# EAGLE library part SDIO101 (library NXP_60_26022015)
SD/SDIO/MMC/CE-ATA host controller The SDIO101 is a SD/SDIO/MMC/CE-ATA host controller with a standard 16-bit asynchronous memory interface. The device conforms to the SD Host Standard Specification Version 2.0. The SDIO101 manages the physical layer of SD, SDIO, MMC and CE-ATA protocols and can be used together with SD Host Standard compatible driver software to add SD/SDIO/MMC/CE-ATA host functionality to a variety of microprocessor systems. The SDIO101 supports both full-speed (lower than 25 MHz) and high-speed (lower than 52 MHz) data transmissions on the SD/SDIO/MMC/CE-ATA port. The SDIO101 offers separate pins for SD/SDIO/MMC/CE-ATA port supply voltage, host interface supply voltage and core supply voltage. The SD/SDIO/MMC/CE-ATA port can operate at a wide voltage range (1.8 V to 3.6 V) which allows the device to interface to a large variety of SD, SDIO, MMC or CE-ATA devices. The SDIO101 allows 1-bit and 4-bit SD transactions and 8-bit MMC/CE-ATA transactions. The 16-bit asynchronous memory interface can operate at a 2.5 V to 3.6 V voltage range. A built-in, 2 kB data buffer allows for a low interrupt latency time and efficient communication with the host processor at high data rates. The SDIO101 provides a DMA request line that can be connected to an external DMA controller to off-load the host processor and increase overall system performance. An on-board PLL allows a large range of SD/SDIO/MMC/CE-ATA clock speeds to be generated from a single externally available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
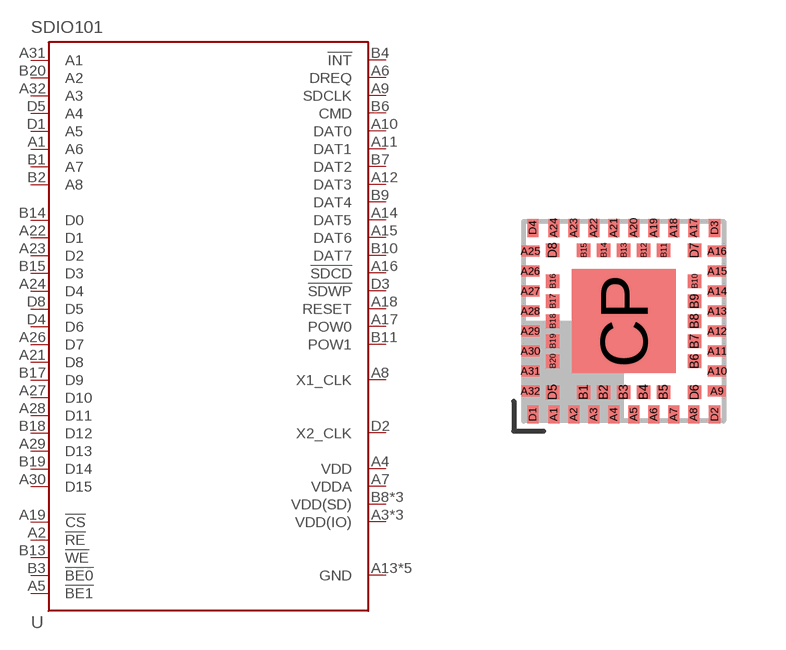
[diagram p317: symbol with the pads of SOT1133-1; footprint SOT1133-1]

Designator prefix U

## SDIO101  [SOT1133-1]
A1  A6  in
A2  !RE  in
A3  VDD(IO)  pwr
A4  VDD  pwr
A5  !BE1  in
A6  DREQ  out
A7  VDDA  pwr
A8  X1_CLK  in
A9  SDCLK
A10  DAT0
A11  DAT1
A12  DAT3
A13  GND  pwr
A14  DAT5
A15  DAT6
A16  !SDCD  in
A17  POW0  out
A18  RESET  in
A19  !CS  in
A20  GND  pwr
A21  D8
A22  D1
A23  D2
A24  D4
A25  GND  pwr
A26  D7
A27  D10
A28  D11
A29  D13
A30  D15
A31  A1  in
A32  A3  in
B1  A7  in
B2  A8  in
B3  !BE0  in
B4  !INT  out
B5  GND  pwr
B6  CMD
B7  DAT2
B8  VDD(SD)  pwr
B9  DAT4
B10  DAT7
B11  POW1  out
B12  VDD(IO)  pwr
B13  !WE  in
B14  D0
B15  D3
B16  VDD(IO)  pwr
B17  D9
B18  D12
B19  D14
B20  A2  in
CP  GND  pwr
D1  A5  in
D2  X2_CLK  out
D3  !SDWP  in
D4  D6
D5  A4  in
D6  VDD(SD)  pwr
D7  VDD(SD)  pwr
D8  D5

## Footprint SOT1133-1 (pad centres in mm)
SOT1133-1 HXQFN60U: plastic thermal enhanced extremely thin quad flat package; no leads; 60 terminals; UTLP based; body 5 x 5 x 0.5 mm JEDEC: -- IEC: -- JEITA: --
smd 0.275 x 0.45: A1 -1.75,-2.335; A2 -1.25,-2.335; A3 -0.75,-2.335; A4 -0.25,-2.335; A5 0.25,-2.335; A6 0.75,-2.335; A7 1.25,-2.335; A8 1.75,-2.335; A17 1.75,2.335; A18 1.25,2.335; A19 0.75,2.335; A20 0.25,2.335; A21 -0.25,2.335; A22 -0.75,2.335; A23 -1.25,2.335; A24 -1.75,2.335; D1 -2.275,-2.335; D2 2.275,-2.335; D3 2.275,2.335; D4 -2.275,2.335
smd 0.45 x 0.275: A9 2.335,-1.75; A10 2.335,-1.25; A11 2.335,-0.75; A12 2.335,-0.25; A13 2.335,0.25; A14 2.335,0.75; A15 2.335,1.25; A16 2.335,1.75; A25 -2.335,1.75; A26 -2.335,1.25; A27 -2.335,0.75; A28 -2.335,0.25; A29 -2.335,-0.25; A30 -2.335,-0.75; A31 -2.335,-1.25; A32 -2.335,-1.75
smd 0.33 x 0.33: B1 -1,-1.775; B2 -0.5,-1.775; B3 0,-1.775; B4 0.5,-1.775; B5 1,-1.775; B6 1.775,-1; B7 1.775,-0.5; B8 1.775,0; B9 1.775,0.5; B10 1.775,1; B11 1,1.775; B12 0.5,1.775; B13 0,1.775; B14 -0.5,1.775; B15 -1,1.775; B16 -1.775,1; B17 -1.775,0.5; B18 -1.775,0; B19 -1.775,-0.5; B20 -1.775,-1; D5 -1.775,-1.775; D6 1.775,-1.775; D7 1.775,1.775; D8 -1.775,1.775
smd 2.6 x 2.6: CP 0,0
